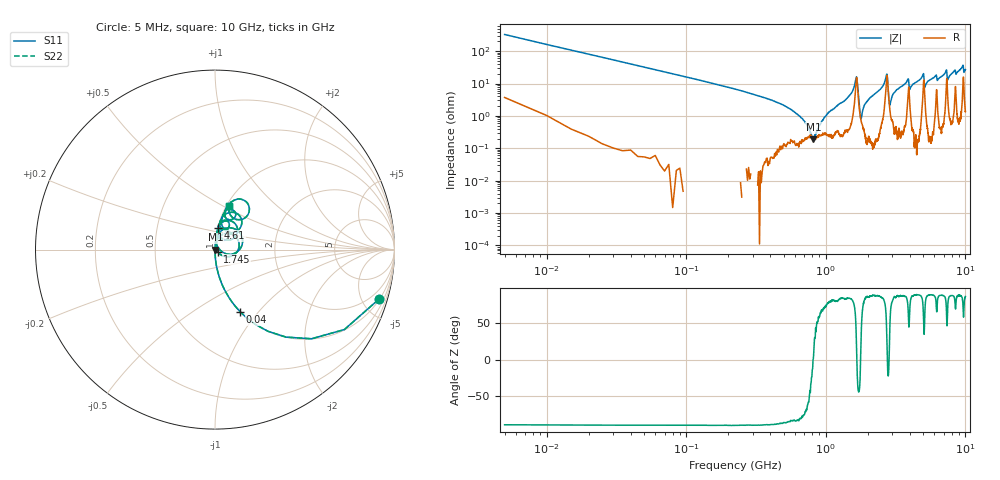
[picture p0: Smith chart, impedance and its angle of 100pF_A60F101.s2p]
! Amotech Co.,Ltd.
! http://www.amotech.co.kr/
! Part Number: A60F101
! These Parameters are Measured in Series Mode Connection
! Operation Temp=25[degC], DC Bias Voltage=0[V]
! Freq. Start=5[MHz] Stop=10[GHz], 2000[Steps]
! Date: Monday, July 20, 2020, 03:44:11
# GHZ S RI R 50.000000
!Freq.(Hz) S11(Real) S11(Imag) S21(Real) S21(Imag) S12(Real) S12(Imag) S22(Real) S22(Imag)
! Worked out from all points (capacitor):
!   2000 points, 5 MHz to 10 GHz, reference 50 ohm
!   read as one part in series: C = 98.5 pF near 55 MHz
!   lowest |Z| = 189 mohm at 815 MHz (marker M1)
!   series resonance near 810.1 MHz, so ESL is about 390 pH
!   S11 on the Smith chart (normalised r, x): 5 MHz: 1.07, -6.56; 40 MHz: 1.00, -0.81; 1.745 GHz: 1.03, -0.02; 4.61 GHz: 1.00, +0.25; 10 GHz: 1.03, +0.54
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0.005  0.9123 -0.2772  0.0877 0.2772  0.0877 0.2772  0.9123 -0.2772
0.04  0.1402 -0.3461  0.8598 0.3461  0.8598 0.3461  0.1402 -0.3461
0.08  0.0385 -0.1925  0.9615 0.1925  0.9615 0.1925  0.0385 -0.1925
0.17  0.00805 -0.091  0.9919 0.091  0.9919 0.091  0.00805 -0.091
0.605  0.00144 -0.0124  0.9986 0.0124  0.9986 0.0124  0.00144 -0.0124
0.815  0.00188 7.58e-05  0.9981 -7.58e-05  0.9981 -7.58e-05  0.00188 7.58e-05
1.05  0.0026 0.0125  0.9974 -0.0125  0.9974 -0.0125  0.0026 0.0125
1.675  0.1133 -0.0234  0.8867 0.0234  0.8867 0.0234  0.1133 -0.0234
1.745  0.0141 -0.0111  0.9859 0.0111  0.9859 0.0111  0.0141 -0.0111
1.805  0.00599 0.00744  0.994 -0.00744  0.994 -0.00744  0.00599 0.00744
1.96  0.00207 0.0265  0.9979 -0.0265  0.9979 -0.0265  0.00207 0.0265
2.71  0.1016 0.1183  0.8984 -0.1183  0.8984 -0.1183  0.1016 0.1183
2.88  0.0148 0.016  0.9852 -0.016  0.9852 -0.016  0.0148 0.016
3.34  0.00917 0.0703  0.9908 -0.0703  0.9908 -0.0703  0.00917 0.0703
4.61  0.0164 0.1203  0.9836 -0.1203  0.9836 -0.1203  0.0164 0.1203
5.005  0.1137 0.1421  0.8863 -0.1421  0.8863 -0.1421  0.1137 0.1421
5.13  0.0335 0.0674  0.9665 -0.0674  0.9665 -0.0674  0.0335 0.0674
6.67  0.0292 0.1554  0.9708 -0.1554  0.9708 -0.1554  0.0292 0.1554
7.295  0.1178 0.2034  0.8822 -0.2034  0.8822 -0.2034  0.1178 0.2034
7.46  0.0552 0.109  0.9448 -0.109  0.9448 -0.109  0.0552 0.109
8.335  0.0735 0.2252  0.9265 -0.2252  0.9265 -0.2252  0.0735 0.2252
10  0.0785 0.2449  0.9215 -0.2449  0.9215 -0.2449  0.0785 0.2449
